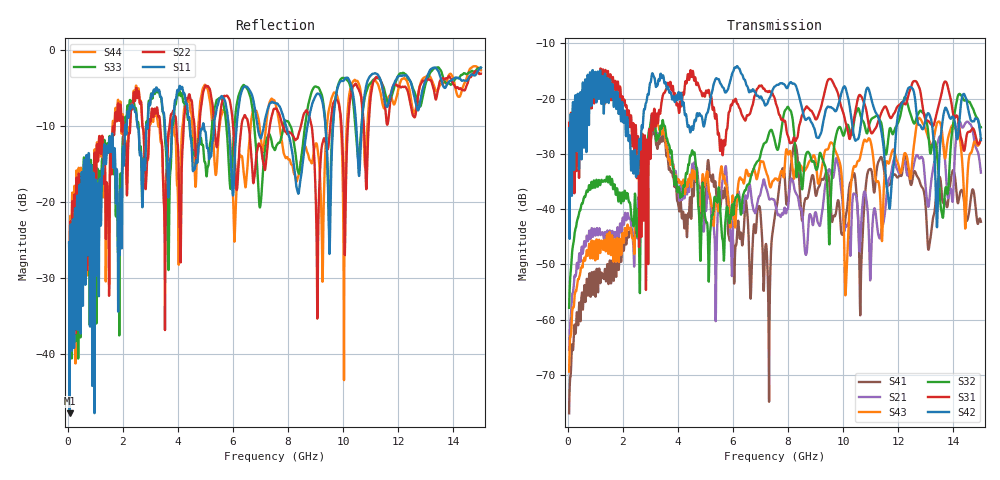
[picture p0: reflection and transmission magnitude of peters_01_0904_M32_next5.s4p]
# MHZ S RI R 50.00
! FREQ  S11  S12  S13  S14
!  S21  S22  S23  S24
!  S31  S32  S33  S34
!  S41  S42  S43  S44
!  REAL  IMAG  REAL  IMAG  REAL  IMAG  REAL  IMAG
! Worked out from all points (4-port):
!   1496 points, 50 MHz to 15 GHz, reference 50 ohm
!   strongest paths, dB at 50 MHz, 3.79 GHz, 7.53 GHz, 11.27 GHz, 15 GHz:
!     S42: -25.4, -20.1, -17.8, -23.3, -27.5
!     S31: -24.4, -18.2, -20.3, -24.2, -27.3
!     S32: -57.9, -30.9, -28.0, -23.3, -25.2
!     S43: -69.4, -31.4, -34.5, -35.0, -27.3
!     S21: -65.4, -31.6, -39.0, -44.5, -33.4
!     S41: -76.9, -33.4, -40.9, -31.6, -42.3
!   lowest |S11| = -47.8 dB at 70 MHz (marker M1), VSWR 1.01, Z = 50.3 - j0.26 ohm
!   |S11| at or under -10 dB: start of sweep to 2.088 GHz; 4.434 GHz to 4.899 GHz (465.1 MHz wide, 9.97 % of centre); 7.915 GHz to 8.706 GHz (791.5 MHz wide, 9.52 % of centre)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
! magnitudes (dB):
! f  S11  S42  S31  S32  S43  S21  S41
! 50 MHz  -25.3  -25.4  -24.4  -57.9  -69.4  -65.4  -76.9
! 70 MHz  -47.8  -45.4  -35.1  -54.5  -65.0  -62.3  -72.4
! 3.1 GHz  -5.7  -15.7  -25.4  -23.2  -23.2  -24.7  -25.5
! 5.13 GHz  -14.4  -21.5  -18.6  -51.4  -37.0  -37.4  -32.4
! 9.59 GHz  -13.2  -21.7  -16.7  -34.0  -28.0  -34.0  -42.2
! 10.11 GHz  -3.7  -18.5  -24.7  -25.2  -52.9  -43.1  -40.9
! 15 GHz  -2.4  -27.5  -27.3  -25.2  -27.3  -33.4  -42.3
